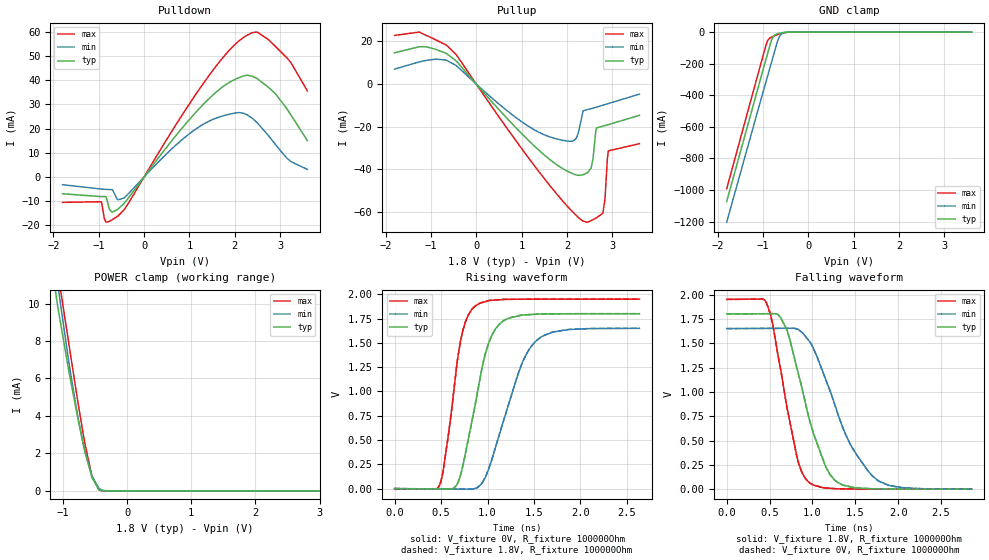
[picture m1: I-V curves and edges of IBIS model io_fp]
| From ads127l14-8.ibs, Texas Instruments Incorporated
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|   io_fp Model
[Model]   io_fp
Model_type   I/O
Polarity   Non-Inverting
Enable   Active-Low
Vinl = 0.54
Vinh = 1.26
Vmeas = 0.9
Vref = 0
Cref = 2pF
Rref = 100000
|   typ   min   max
C_comp   0.482pF   0.525pF   0.457pF
[Voltage Range]   1.8   1.65   1.95
[Temperature Range]   27   125   -40
[Pullup Reference]   1.8   1.65   1.95
[Pulldown Reference]   0   0   0
[Power Clamp Reference]   1.8   1.65   1.95
[GND Clamp Reference]   0   0   0
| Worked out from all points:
|   slope of the pulldown table from 0 to 0.27 V, typ, clamps not added: 39.9 ohm
|   slope of the pullup table from 0 to 0.27 V, typ, clamps not added: 41.3 ohm
|   GND clamp passes 1 mA (typ) near -0.47 V on its own axis
|   POWER clamp passes 1 mA (typ) near -0.57 V on its own axis
|   falling waveform, V_fixture 1.8V, R_fixture 100000Ohm: 20-80 % time 335ps typ, 463ps min, 243ps max; typ from 1.8 V to 0.001 V
|   rising waveform, V_fixture 0V, R_fixture 100000Ohm: 20-80 % time 231ps typ, 329ps min, 164ps max; typ from 0 V to 1.8 V
|   rising waveform, V_fixture 1.8V, R_fixture 100000Ohm: 20-80 % time 231ps typ, 329ps min, 164ps max; typ from 0.001 V to 1.8 V
|   falling waveform, V_fixture 0V, R_fixture 100000Ohm: 20-80 % time 335ps typ, 462ps min, 243ps max; typ from 1.8 V to 0 V
[Pulldown]
|   Voltage   I(typ)   I(min)   I(max)
-1.8V     -6.966mA   -3.237mA   -10.54mA
-946.8mV  -8.148mA   -5.018mA   -10.27mA
-844.2mV  -8.107mA   -5.157mA   -18.59mA
-714.6mV  -14.52mA   -5.288mA   -17.82mA
-579.6mV  -13.39mA   -9.491mA   -16.24mA
-444.6mV  -11.02mA   -8.752mA   -13.66mA
1.262V    29.17mA    21.31mA    37.49mA
2.05V     40.74mA    26.54mA    55.59mA
2.38V     41.74mA    24.35mA    59.66mA
2.741V    37.12mA    17.11mA    56.81mA
3.136V    28.54mA    8.018mA    49.53mA
3.6V      15.03mA    3.097mA    35.59mA
[GND Clamp]
|   Voltage   I(typ)   I(min)   I(max)
-1.8V     -1.073A    -1.203A    -991.6mA
-1.071V   -314.6mA   -454.1mA   -226.3mA
-909mV    -148.1mA   -289.9mA   -62.57mA
-865.8mV  -104.2mA   -246.2mA   -42.09mA
-811.8mV  -51.93mA   -191.7mA   -31.97mA
-768.6mV  -27.22mA   -148.2mA   -26.46mA
-671.4mV  -10.31mA   -52.75mA   -15.22mA
-633.6mV  -7.434mA   -27.57mA   -11.39mA
-590.4mV  -4.838mA   -11.77mA   -7.591mA
-536.4mV  -2.477mA   -3.932mA   -3.947mA
-369mV    -68.86uA   -116.7uA   -98.27uA
3.6V      0A         0A         0A
[Pullup]
|   Voltage   I(typ)   I(min)   I(max)
-1.8V     14.68mA    7.012mA    22.83mA
-1.26V    17.48mA    10.37mA    24.39mA
-444.6mV  10.94mA    8.719mA    13.9mA
1.597V    -35mA      -24.62mA   -46.94mA
2.18V     -42.53mA   -26.12mA   -61.16mA
2.358V    -42.6mA    -12.54mA   -64.4mA
2.536V    -39.25mA   -11.54mA   -64.16mA
2.655V    -20.6mA    -10.85mA   -62.81mA
2.795V    -19.76mA   -9.933mA   -60.42mA
2.839V    -19.51mA   -9.652mA   -54.3mA
2.914V    -19.08mA   -9.165mA   -31.39mA
3.6V      -14.68mA   -4.746mA   -28.02mA
[POWER Clamp]
|   Voltage   I(typ)   I(min)   I(max)
-1.8V     31.21mA    30.7mA     34.75mA
-1.103V   10.28mA    11.52mA    12.12mA
-1.082V   9.797mA    10.98mA    11.66mA
-914.4mV  6.469mA    6.968mA    7.947mA
-774mV    3.948mA    4.022mA    4.833mA
-687.6mV  2.529mA    2.527mA    3.066mA
-655.2mV  2.04mA     2.046mA    2.454mA
-547.2mV  695.3uA    782.9uA    771uA
-439.2mV  77.92uA    141.2uA    59.87uA
-374.4mV  11.15uA    32.03uA    6.079uA
-261mV    174.7nA    1.497uA    51.88nA
3.6V      0A         0A         0A
[Ramp]
R_load = 100000
|   typ   min   max
dV/dt_r   1.07956/2.30213e-10   0.989492/3.28657e-10   1.16963/1.63865e-10
dV/dt_f   1.07958/3.35622e-10   0.989512/4.61896e-10   1.16963/2.41808e-10
[Falling Waveform]
V_fixture = 1.8V
V_fixture_min = 1.65V
V_fixture_max = 1.95V
R_fixture = 100000Ohm
C_fixture = 0F
|   Time   V(typ)   V(min)   V(max)
0s        1.8V       1.65V      1.95V
462.6ps   1.803V     1.652V     1.917V
534.9ps   1.803V     1.653V     1.704V
698.8ps   1.643V     1.653V     861.2mV
839.4ps   1.173V     1.638V     266.5mV
965.1ps   714.6mV    1.519V     66.74mV
1.256ns   96.1mV     880.6mV    6.161mV
1.435ns   26.2mV     473.4mV    2.372mV
1.7ns     3.81mV     135.3mV    816.9uV
2.855ns   815.5uV    930.2uV    681.9uV
[Rising Waveform]
V_fixture = 0V
V_fixture_min = 0V
V_fixture_max = 0V
R_fixture = 100000Ohm
C_fixture = 0F
|   Time   V(typ)   V(min)   V(max)
0s        1.403nV    17.93nV    12.01nV
485.3ps   -3.454mV   -2.947mV   40.26mV
527.5ps   -3.754mV   -3.204mV   213.9mV
714ps     153.4mV    -4.337mV   1.54V
868.3ps   870.7mV    2.055mV    1.879V
980.2ps   1.4V       125.2mV    1.924V
1.088ns   1.646V     431.4mV    1.94V
1.374ns   1.785V     1.296V     1.948V
1.517ns   1.793V     1.515V     1.949V
2.634ns   1.799V     1.649V     1.949V
[Rising Waveform]
V_fixture = 1.8V
V_fixture_min = 1.65V
V_fixture_max = 1.95V
R_fixture = 100000Ohm
C_fixture = 0F
|   Time   V(typ)   V(min)   V(max)
0s        706.9uV    813.3uV    614.2uV
485.3ps   -2.734mV   -2.114mV   40.92mV
527.5ps   -3.034mV   -2.369mV   214.6mV
714ps     154.3mV    -3.494mV   1.541V
868.3ps   871.9mV    2.935mV    1.879V
980.2ps   1.401V     127.8mV    1.927V
1.088ns   1.646V     431.8mV    1.941V
1.366ns   1.785V     1.278V     1.949V
1.51ns    1.794V     1.509V     1.95V
2.634ns   1.8V       1.65V      1.95V
[Falling Waveform]
|Gnd
V_fixture = 0V
V_fixture_min = 0V
V_fixture_max = 0V
R_fixture = 100000Ohm
C_fixture = 0F
|   Time   V(typ)   V(min)   V(max)
0s        1.799V     1.649V     1.949V
462.6ps   1.802V     1.651V     1.916V
534.9ps   1.803V     1.652V     1.703V
698.8ps   1.642V     1.652V     860.3mV
839.4ps   1.172V     1.637V     265.6mV
961.6ps   724.5mV    1.522V     68.5mV
1.256ns   95.22mV    879.1mV    5.542mV
1.445ns   23.49mV    455mV      1.697mV
1.7ns     3.098mV    134mV      202.6uV
2.855ns   108.4uV    116.5uV    67.76uV
